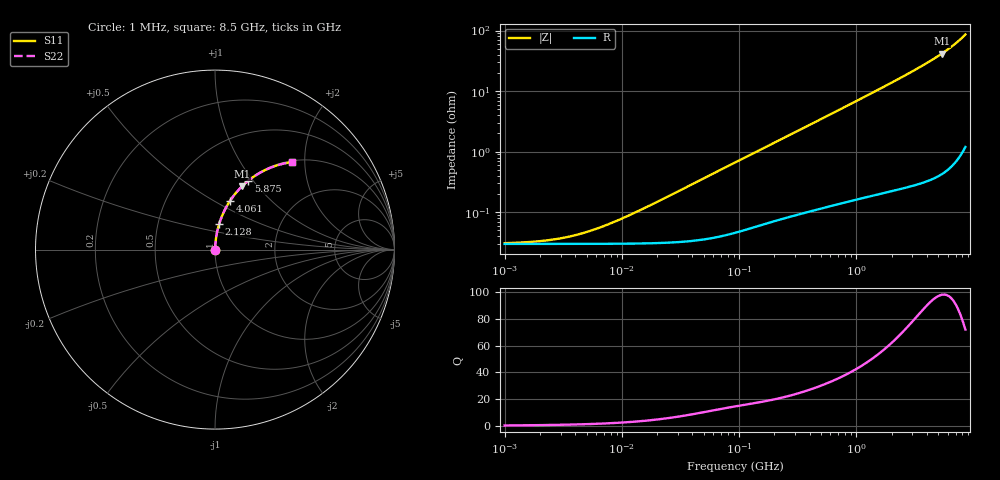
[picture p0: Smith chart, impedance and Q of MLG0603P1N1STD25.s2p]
! S-Parameter Data Generated by TDK Corporation
! Copyright(C) 2025 TDK Corporation.
! All Rights Reserved.
! TDK P/N: MLG0603P1N1STD25 (SMD / SMT Inductor (Coil))
! Property: L=1.1nH at 500MHz
! Size(LxWxT): 0.6x0.3x0.3mm
! Model Type: s2p (Touchstone File Format Version 1.0)
! Frequency: DC=Yes Start=1MHz Stop=8500MHz 198points Log-sweep
! Model Generated on Feb. 6, 2025
! Terms and conditions regarding TDK Simulation Models:
! 1)This simulation model is being provided solely for informational
!  purposes. Please refer to the specifications of the products in
!  terms of detailed characteristics of such products.
! 2)In no event shall TDK Corporation of any of its subsidiaries be
!  liable for any loss or damage arising, directly or indirectly,
!  from any information contained in this simulation model, including,
!  but not limited to loss or damages arising from any inaccuracies,
!  omissions or errors in connection with such information.
! 3)Any and all copyrights on this simulation model are owned by
!  TDK Corporation.  Duplication or redistribution of this simulation
!  model without prior written permission from TDK Corporation
!  is prohibited.
! 4)This simulation model is subject to any modification or change
!  without any prior notice.
! 5)Neither TDK Corporation nor any of its subsidiaries shall make any
!  warranty, express or implied, including but not limited to the
!  correctness, implied warranties of merchantability and fitness for
!  a particular purpose with respect to this simulation models.
! 6)The use of this simulation model shall be deemed to have consented
!  to the terms and conditions hereof.
! Port Assignments:
!  1 ---@@@--- 2
! Applicable Conditions:
!  Temperature = 25 degC
!  DC Bias Current = 0 A
!  Small Signal Operation
# Hz S MA R 50
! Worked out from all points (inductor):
!   197 points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, 1 MHz to 8.5 GHz, reference 50 ohm
!   read as one part in series: L = 1.16 nH near 12.67 MHz
!   highest Q = 98 at 5.357 GHz (marker M1), where L = 1.24 nH
!   S11 on the Smith chart (normalised r, x): 1 MHz: 1.00, +0.00; 2.128 GHz: 1.00, +0.29; 4.061 GHz: 1.01, +0.59; 5.875 GHz: 1.01, +0.94; 8.5 GHz: 1.02, +1.72
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1000000  0.0003086 13.6  0.9997 -0.0  0.9997 -0.0  0.0003086 13.6
1586648  0.0003213 21.0  0.9997 -0.0  0.9997 -0.0  0.0003213 21.0
2403882  0.0003472 30.2  0.9997 -0.0  0.9997 -0.0  0.0003472 30.2
3320851  0.0003851 38.8  0.9997 -0.0  0.9997 -0.0  0.0003851 38.8
4587603  0.0004486 47.9  0.9997 -0.0  0.9997 -0.0  0.0004486 47.9
6337562  0.0005499 56.8  0.9997 -0.0  0.9997 -0.0  0.0005499 56.8
8755050  0.0007038 64.6  0.9997 -0.0  0.9997 -0.0  0.0007038 64.6
1.26661e7  0.0009686 71.7  0.9997 -0.1  0.9997 -0.1  0.0009686 71.7
2.10461e7  0.001559 78.4  0.9997 -0.1  0.9997 -0.1  0.001559 78.4
9.219544e7  0.006626 85.7  0.9995 -0.4  0.9995 -0.4  0.006626 85.7
4.229561e8  0.02928 86.3  0.9985 -1.7  0.9985 -1.7  0.02928 86.3
1.016736e9  0.06954 84.7  0.996 -4.0  0.996 -4.0  0.06954 84.7
1.940355e9  0.1326 81.4  0.989 -7.6  0.989 -7.6  0.1326 81.4
2.128028e9  0.1456 80.7  0.9871 -8.4  0.9871 -8.4  0.1456 80.7
3.07866e9  0.2124 77.0  0.9745 -12.3  0.9745 -12.3  0.2124 77.0
4.061159e9  0.2841 72.9  0.9557 -16.5  0.9557 -16.5  0.2841 72.9
4.664383e9  0.3297 70.2  0.9406 -19.2  0.9406 -19.2  0.3297 70.2
5.357206e9  0.3837 66.9  0.9195 -22.6  0.9195 -22.6  0.3837 66.9
5.87536e9  0.4254 64.2  0.9007 -25.2  0.9007 -25.2  0.4254 64.2
7.066863e9  0.5247 57.7  0.8455 -31.6  0.8455 -31.6  0.5247 57.7
7.750377e9  0.5836 53.6  0.805 -35.7  0.805 -35.7  0.5836 53.6
8.5e9  0.6486 48.8  0.7521 -40.4  0.7521 -40.4  0.6486 48.8
